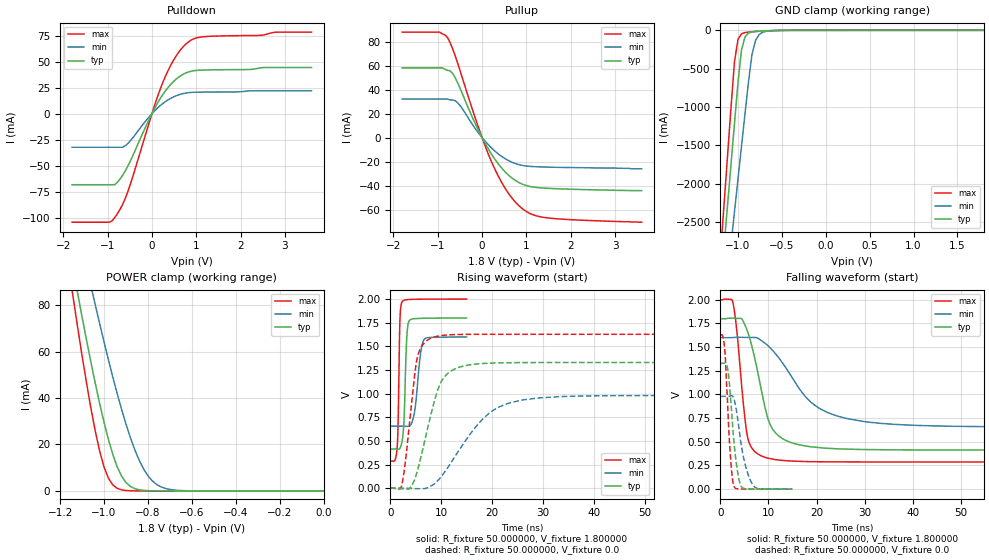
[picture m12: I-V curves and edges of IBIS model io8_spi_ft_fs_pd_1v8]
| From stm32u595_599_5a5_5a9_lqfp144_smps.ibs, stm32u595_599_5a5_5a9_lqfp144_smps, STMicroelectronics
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|   Model io8_spi_ft_fs_pd_1v8
[Model]  io8_spi_ft_fs_pd_1v8
Model_type I/O
Polarity   Non-Inverting
Enable   Active-Low
Vinl =   0.540000V
Vinh =   1.260000V
Vmeas =  0.900000V
Cref =   50.000000pF
Rref =   100.000000M
Vref =   0.0V
C_comp   3.338500pF   3.332300pF   3.378900pF
[Temperature Range]   25.000000   0.140000k   -40.000000
[Pullup Reference]   1.800000V   1.600000V   2.000000V
[Pulldown Reference]   0.0V   0.0V   0.0V
[POWER Clamp Reference]   1.800000V   1.600000V   2.000000V
[GND Clamp Reference]   0.0V   0.0V   0.0V
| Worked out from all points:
|   slope of the pulldown table from 0 to 0.27 V, typ, clamps not added: 13.6 ohm
|   slope of the pullup table from 0 to 0.27 V, typ, clamps not added: 15.9 ohm
|   GND clamp passes 1 mA (typ) near -0.50 V on its own axis
|   POWER clamp passes 1 mA (typ) near -0.86 V on its own axis
|   rising waveform, R_fixture 50.000000, V_fixture 1.800000: 20-80 % time 508ps typ, 1.05ns min, 328ps max; typ from 0.414 V to 1.8 V
|   rising waveform, R_fixture 50.000000, V_fixture 0.0: 20-80 % time 3.76ns typ, 8.23ns min, 1.98ns max; typ from 0 V to 1.33 V
|   falling waveform, R_fixture 50.000000, V_fixture 1.800000: 20-80 % time 3.8ns typ, 9.16ns min, 1.95ns max; typ from 1.8 V to 0.414 V
|   falling waveform, R_fixture 50.000000, V_fixture 0.0: 20-80 % time 1.37ns typ, 2.02ns min, 1ns max; typ from 1.33 V to 0 V
[Pulldown]
|Voltage   I(typ)   I(min)   I(max)
-1.8V     -68.38mA   -32.32mA   -104.4mA
-960mV    -68.38mA   -32.32mA   -104.4mA
-780mV    -66.07mA   -32.32mA   -96.42mA
-660mV    -59.2mA    -32.31mA   -87.22mA
-540mV    -50.22mA   -28.51mA   -74.66mA
0V        -10fA      -300fA     0A
240mV     18.04mA    9.599mA    29.41mA
480mV     30.68mA    16.02mA    50.95mA
780mV     39.47mA    19.98mA    67.56mA
960mV     41.44mA    20.62mA    72.37mA
1.14V     41.99mA    20.78mA    74.01mA
3.6V      44.44mA    22.06mA    78.55mA
[Pullup]
|Voltage   I(typ)   I(min)   I(max)
-1.8V     58.04mA    32.12mA    87.86mA
-960mV    58.04mA    32.12mA    87.86mA
-780mV    55.99mA    32.12mA    83.36mA
-660mV    53.21mA    31.28mA    73.65mA
-540mV    44.81mA    28.64mA    60.84mA
-120mV    9.014mA    5.781mA    12.75mA
240mV     -15.38mA   -9.6mA     -22.37mA
540mV     -29.31mA   -18.02mA   -43.36mA
900mV     -38.69mA   -23.13mA   -58.99mA
1.14V     -41.14mA   -24.16mA   -64.17mA
1.5V      -42.31mA   -24.64mA   -67mA
3.6V      -44.2mA    -26mA      -70.5mA
[GND_clamp]
|Voltage   I(typ)   I(min)   I(max)
-1.8V     -9.908A    -9.683A    -9.994A
-1.2V     -3.383A    -4.084A    -2.934A
-1.16V    -2.841A    -3.655A    -2.294A
-1.12V    -2.299A    -3.226A    -1.656A
-1.04V    -1.218A    -2.369A    -414.2mA
-1V       -684.7mA   -1.941A    -119.2mA
-960mV    -257.2mA   -1.514A    -45.67mA
-920mV    -87.04mA   -1.089A    -28.94mA
-840mV    -19.36mA   -312.8mA   -18.98mA
-800mV    -13.56mA   -132.4mA   -15.51mA
-720mV    -8.053mA   -25.67mA   -9.504mA
1.8V      45.71uA    33.32uA    56.11uA
[POWER_clamp]
|Voltage   I(typ)   I(min)   I(max)
-1.8V     470.8mA    433.7mA    554.6mA
-1.14V    95.25mA    122.7mA    82.82mA
-1.12V    84.97mA    114mA      70.27mA
-1.06V    55.51mA    88.42mA    35.67mA
-1.04V    46.34mA    80.15mA    25.76mA
-1V       29.51mA    64.13mA    10.3mA
-940mV    10.39mA    41.86mA    1.109mA
-900mV    3.624mA    28.77mA    182.8uA
-840mV    490.7uA    13.24mA    11.35uA
-800mV    116.8uA    6.532mA    1.77uA
-740mV    13.2uA     1.724mA    109.3nA
0V        0A         18.75nA    0A
[Ramp]
| variable   typ   min   max
dV/dt_r  0.79740/3.76096n   0.58784/8.22044n   0.97632/1.97598n
dV/dt_f  0.83141/3.79765n   0.56582/9.14498n   1.02743/1.94048n
R_load = 50.000000
[Rising Waveform]
R_fixture= 50.000000
V_fixture= 1.800000
V_fixture_min= 1.600000
V_fixture_max= 2.000000
|time   V(typ)   V(min)   V(max)
0s        413.8mV    656.5mV    287.1mV
1.381ns   412.9mV    656.5mV    452.7mV
1.892ns   422.8mV    656.5mV    1.771V
2.282ns   488.3mV    656.5mV    1.966V
2.703ns   734.1mV    656.3mV    1.988V
3.243ns   1.597V     654.8mV    1.993V
3.694ns   1.768V     655.6mV    1.995V
4.745ns   1.793V     804mV      1.997V
6.667ns   1.797V     1.575V     1.998V
14.95ns   1.8V       1.599V     2V
[Rising Waveform]
R_fixture= 50.000000
V_fixture= 0.0
V_fixture_min= 0.0
V_fixture_max= 0.0
|time   V(typ)   V(min)   V(max)
0s        2.135uV    2.367uV    264.9nV
2.202ns   -3.958mV   1.958uV    20.56mV
4.404ns   46.45mV    -3.235mV   1.01V
5.606ns   242.3mV    -4.855mV   1.437V
8.609ns   911.4mV    44.53mV    1.598V
10.21ns   1.146V     138.9mV    1.615V
12.61ns   1.26V      328.9mV    1.624V
19.22ns   1.321V     784.6mV    1.627V
25.83ns   1.328V     932.1mV    1.627V
99.7ns    1.329V     979.8mV    1.627V
[Falling Waveform]
R_fixture= 50.000000
V_fixture= 1.800000
V_fixture_min= 1.600000
V_fixture_max= 2.000000
|time   V(typ)   V(min)   V(max)
0s        1.8V       1.599V     2V
2.603ns   1.805V     1.6V       1.973V
3.403ns   1.803V     1.603V     1.676V
5.606ns   1.67V      1.602V     560.9mV
9.009ns   925.6mV    1.551V     340.8mV
10.61ns   655.7mV    1.478V     320mV
13.01ns   530.8mV    1.325V     302.8mV
18.82ns   447.6mV    919.1mV    290.5mV
26.43ns   422.6mV    744mV      287.6mV
99.7ns    413.8mV    656.5mV    287.1mV
[Falling Waveform]
R_fixture= 50.000000
V_fixture= 0.0
V_fixture_min= 0.0
V_fixture_max= 0.0
|time   V(typ)   V(min)   V(max)
0s        1.329V     979.8mV    1.627V
510.5ps   1.329V     979.8mV    1.611V
930.9ps   1.334V     979.8mV    1.461V
1.562ns   1.254V     979.7mV    828.3mV
2.162ns   926.8mV    985.7mV    295.7mV
2.853ns   479.6mV    945.3mV    26.41mV
4.174ns   46.82mV    523mV      1.924mV
5.135ns   5.62mV     263.9mV    967.8uV
6.607ns   1.703mV    56.08mV    521.6uV
14.95ns   2.135uV    2.367uV    264.9nV
